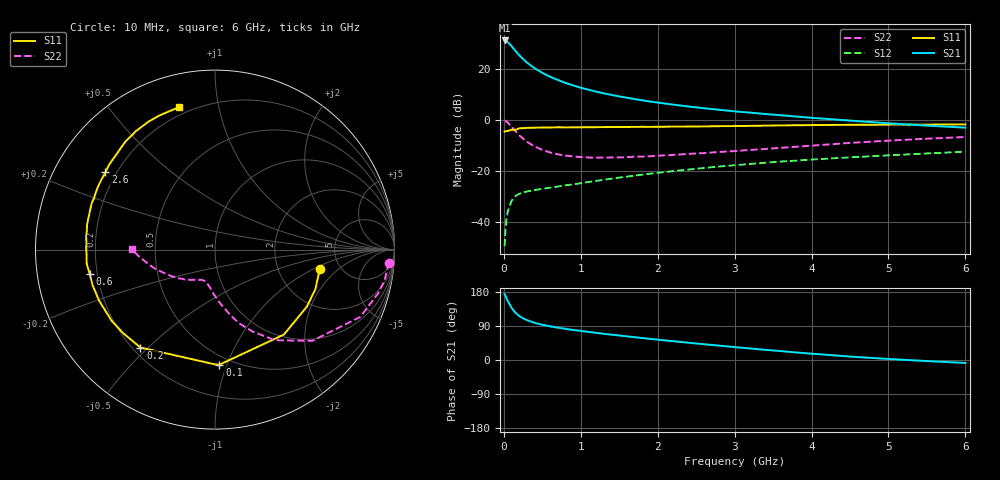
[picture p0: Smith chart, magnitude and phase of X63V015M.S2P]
! SIEMENS Small Signal Semiconductors
! BFP193W
! Si NPN RF Bipolar Junction Transistor in SOT343
! VCE = 3 V  IC = 15 mA
! Common Emitter S-Parameters:  April 1994
# GHz  S  MA  R  50
!  f  S11  S21  S12  S22
! GHz  MAG  ANG  MAG  ANG  MAG  ANG  MAG  ANG
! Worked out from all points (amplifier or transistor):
!   40 points, 10 MHz to 6 GHz, reference 50 ohm
!   highest |S21| = 31.1 dB at 10 MHz (marker M1)
!   |S21| within 3 dB of that: start of sweep to 120.7 MHz
!   unconditionally stable (mu >= 1): 1.069 GHz to 4.113 GHz
!   at 200 MHz: K = 0.29, MSG = 27.1 dB, |S12| = -28.9 dB
!   at 1.5 GHz: K = 1.10, MAG = 13.9 dB, |S12| = -22.6 dB
!   at 6 GHz: K = 0.92, MSG = 4.7 dB, |S12| = -12.4 dB
!   S11 on the Smith chart (normalised r, x): 10 MHz: 3.49, -1.19; 100 MHz: 0.43, -0.94; 200 MHz: 0.23, -0.47; 600 MHz: 0.17, -0.09; 2.6 GHz: 0.16, +0.31; 6 GHz: 0.16, +0.76
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0.01  0.5936 -10.7  35.86 174.0  0.0034 86.9  0.9706 -4.3
0.02  0.6014 -21.6  35.7 169.9  0.0068 80.4  0.9606 -10.4
0.03  0.6024 -32.0  35.15 165.1  0.0102 78.9  0.9397 -15.2
0.05  0.6094 -51.0  33.37 155.9  0.0161 69.3  0.8927 -24.8
0.1  0.6418 -87.8  27.69 137.7  0.0263 54.4  0.7429 -43.2
0.15  0.6393 -90.1  22.46 124.8  0.0325 45.5  0.6063 -56.4
0.2  0.6858 -127.3  18.41 116.1  0.0358 40.7  0.5029 -65.3
0.25  0.6919 -137.8  15.51 109.9  0.0382 37.6  0.4311 -72.0
0.3  0.6995 -145.6  13.24 105.3  0.0399 36.4  0.3733 -76.9
0.4  0.7057 -156.3  10.25 98.2  0.0426 35.5  0.3025 -84.3
0.5  0.7104 -163.8  8.336 93.0  0.0449 36.5  0.2595 -89.9
0.6  0.7111 -169.1  7 88.8  0.0474 37.5  0.2311 -94.3
0.8  0.7162 -177.5  5.311 82.2  0.0526 41.1  0.2009 -100.6
1.1  0.7219 174.2  3.906 74.1  0.0611 44.8  0.1843 -107.9
1.3  0.7258 169.3  3.31 69.1  0.0677 47.0  0.1839 -111.6
1.6  0.7296 162.8  2.715 62.3  0.078 49.2  0.1872 -116.3
2.2  0.7402 151.9  1.996 49.6  0.0997 50.5  0.2069 -125.9
2.6  0.7473 144.8  1.696 41.6  0.1149 50.1  0.2248 -132.3
3.2  0.7651 135.2  1.389 30.5  0.1378 48.0  0.2591 -142.0
4.5  0.8033 117.6  0.971 9.1  0.1857 41.2  0.3557 -163.3
5.5  0.8115 108.5  0.775 -2.8  0.2209 35.4  0.4299 -175.5
6  0.8185 104.3  0.707 -7.8  0.2395 32.8  0.4642 179.6
